| Texas Instruments Incorporated
| 1.6-GSPS, 12-bit, Analog-to-Digital Converter
| Marketing part#   ADC12QJ1600AAVQ1
| Voltage Range   1.05V - 1.15V & 1.8V - 2.0V
| Package-type   BGA
| #pins/pkg drawing   144-pin AAV
[IBIS Ver]   4.1
[File name]   adc12qj1600aav.ibs
[File Rev]   1.0
[Date]   12/15/2021
[Source]   Model built from spectre simulations at:
   Texas Instruments Incorporated.
   12500 TI Blvd
   Dallas, TX -75243
   Support: https://e2e.ti.com/support/data-converters/f/data-converters-forum
[Notes]   Rev 1.0: 12/15/2021
[Disclaimer]  This model is designed as an aid for customers of Texas Instruments
 TI and its licensors and suppliers make no warranties, either expressed
 or implied, with respect to this  model, including the warranties of
 merchantability or fitness for a particular purpose.
 The model is provided solely on an "as is" basis. The entire risk as to
 its quality and performance is with the customer.
[Copyright] (C)Copyright 2021 Texas Instruments Incorporated.
   All rights reserved.
[Component]   ADC12QJ1600AAVQ1_PECL   | PECL input on SYNCB, DEVCLK, SYSREF
[Manufacturer]  Texas Instruments Incorporated
[Package]   |144-pin BGA AAV package
|   typ   min   max
R_pkg   0.160   0.009   0.397
L_pkg   1.73E-09   4.81E-10   3.76E-09
C_pkg   7.00E-13   1.77E-13   1.64E-12
[Pin]   signal_name  model_name   R_pin   L_pin   C_pin
A1   AGND   GND
A2   INA+   NC   0.29421   2.39E-09   8.75E-13
A3   INA-   NC   0.29421   2.37E-09   8.77E-13
A4   AGND   GND
A5   AGND   GND
A6   INB+   NC   0.29156   2.27E-09   8.69E-13
A7   INB-   NC   0.29004   2.23E-09   8.66E-13
A8   AGND   GND
A9   CALTRIG   INPUT   0.17604   1.67E-09   5.27E-13
A10   VD11   POWER
A11   DGND   GND
A12   DGND   GND
B1   AGND   GND
B2   AGND   GND
B3   AGND   GND
B4   AGND   GND
B5   AGND   GND
B6   AGND   GND
B7   AGND   GND
B8   AGND   GND
B9   CALSTAT   OUTPUT   0.08157   1.80E-09   1.77E-13
B10   VD11   POWER
B11   DGND   GND
B12   DGND   GND
C1   TMSTP+   SYNCB_PECL   0.39654   3.22E-09   1.10E-12
C2   AGND   GND
C3   BG   NC   0.06662   9.15E-10   6.92E-13
C4   SYNCSE\   INPUT   0.12713   1.23E-09   8.40E-13
C5   AGND   GND
C6   AGND   GND
C7   CLKCFG0   INPUT   0.05783   8.20E-10   6.34E-13
C8   PLLREF_SE   INPUT   0.26767   3.76E-09   8.08E-13
C9   ORA   OUTPUT   0.12512   1.74E-09   4.33E-13
C10   DGND   GND
C11   D7+   NC   0.11238   1.27E-09   5.29E-13
C12   D3+   NC   0.15974   1.68E-09   6.21E-13
D1   TMSTP-   SYNCB_PECL   0.39553   3.09E-09   1.15E-12
D2   AGND   GND
D3   AGND   GND
D4   VA19   POWER
D5   VA19   POWER
D6   VA11   POWER
D7   CLKCFG1   INPUT   0.00903   4.81E-10   5.14E-13
D8   PLL_EN   INPUT   0.16984   2.55E-09   6.19E-13
D9   ORB   OUTPUT   0.05495   1.15E-09   2.51E-13
D10   VD11   POWER
D11   D7-   NC   0.11401   1.31E-09   5.25E-13
D12   D3-   NC   0.16105   1.71E-09   6.11E-13
E1   AGND   GND
E2   AGND   GND
E3   VA11   POWER
E4   AGND   GND
E5   VA11   POWER
E6   VA19   POWER
E7   AGND   GND
E8   SCS\   INPUT_PU   0.12924   1.74E-09   6.18E-13
E9   ORC   OUTPUT   0.17039   2.54E-09   4.96E-13
E10   VD11   POWER
E11   D6+   NC   0.10585   1.24E-09   5.15E-13
E12   D2+   NC   0.17042   1.72E-09   6.38E-13
F1   CLK+   DEVCLK_PECL   0.30857   2.59E-09   1.02E-12
F2   SE_CLK   INPUT   0.05749   1.43E-09   1.64E-12
F3   VA11   POWER
F4   AGND   GND
F5   VA11   POWER
F6   VA19   POWER
F7   AGND   GND
F8   SCLK   INPUT   0.06994   1.23E-09   5.56E-13
F9   ORD   OUTPUT   0.10254   1.74E-09   4.79E-13
F10   DGND   GND
F11   D6-   NC   0.10617   1.32E-09   5.12E-13
F12   D2-   NC   0.17077   1.77E-09   6.34E-13
G1   CLK-   DEVCLK_PECL   0.30912   2.61E-09   1.00E-12
G2   SE_GND   GND   0.05431   1.31E-09   1.58E-12
G3   VA11   POWER
G4   AGND   GND
G5   VA11   POWER
G6   VA19   POWER
G7   AGND   GND
G8   SDI   INPUT   0.04691   9.40E-10   6.68E-13
G9   SDO   OUTPUT   0.1   1.53E-09   5.24E-13
G10   DGND   GND
G11   D5+   NC   0.09799   1.20E-09   4.90E-13
G12   D1+   NC   0.16586   1.74E-09   6.24E-13
H1   AGND   GND
H2   AGND   GND
H3   VA11   POWER
H4   AGND   GND
H5   VA11   POWER
H6   VA19   POWER
H7   AGND   GND
H8   VD11   POWER
H9   VD11   POWER
H10   VD11   POWER
H11   D5-   NC   0.10149   1.24E-09   4.91E-13
H12   D1-   NC   0.16843   1.81E-09   6.24E-13
J1   SYSREF+   SYSREF_PECL   0.29068   2.61E-09   9.76E-13
J2   AGND   GND
J3   PGND   GND
J4   VPLL19   POWER
J5   VPLL19   POWER
J6   VA11   POWER
J7   PLLREFO+   LVDSP_MODE_0_V1P8   0.00902   4.91E-10   4.99E-13
J8   VTRIG   POWER
J9   TRIGOUT+   LVDSP   0.06885   9.55E-10   6.39E-13
J10   VD11   POWER
J11   D4+   NC   0.12851   1.35E-09   5.52E-13
J12   D0+   NC   0.17935   1.78E-09   6.56E-13
K1   SYSREF-   SYSREF_PECL   0.28925   2.55E-09   9.73E-13
K2   AGND   GND
K3   TDIODE+   NC   0.05067   1.14E-09   8.01E-13
K4   TDIODE-   NC   0.04958   1.12E-09   7.88E-13
K5   PGND   GND
K6   VREFO   POWER
K7   PLLREFO-   LVDSN_MODE_0_V1P8   0.00927   5.06E-10   5.46E-13
K8   VTRIG   POWER
K9   TRIGOUT-   LVDSN   0.07317   1.04E-09   6.64E-13
K10   DGND   GND
K11   D4-   NC   0.133   1.46E-09   5.57E-13
K12   D0-   NC   0.18263   1.86E-09   6.52E-13
L1   AGND   GND
L2   AGND   GND
L3   AGND   GND
L4   AGND   GND
L5   AGND   GND
L6   AGND   GND
L7   AGND   GND
L8   AGND   GND
L9   DGND   GND
L10   VD11   POWER
L11   DGND   GND
L12   DGND   GND
M1   AGND   GND
M2   IND+   NC   0.29422   2.39E-09   8.76E-13
M3   IND-   NC   0.29417   2.37E-09   8.75E-13
M4   AGND   GND
M5   AGND   GND
M6   INC+   NC   0.29159   2.49E-09   8.64E-13
M7   INC-   NC   0.29018   2.45E-09   8.64E-13
M8   AGND   GND
M9   PD   INPUT   0.15035   1.56E-09   4.67E-13
M10   VD11   POWER
M11   DGND   GND
M12   DGND   GND
[Diff pin]  inv_pin  vdiff  tdelay_typ  tdelay_min  tdelay_max
A2   A3   0.0   0.0s   0.0s   0.0s   | INA
A6   A7   0.0   0.0s   0.0s   0.0s   | INB
M2   M3   0.0   0.0s   0.0s   0.0s   | IND
M6   M7   0.0   0.0s   0.0s   0.0s   | INC
C1   D1   0.0   0.0s   0.0s   0.0s   | TMSTP
F1   G1   0.0   0.0s   0.0s   0.0s   | CLK
J1   K1   0.0   0.0s   0.0s   0.0s   | SYSREF
J7   K7   0.0   0.0s   0.0s   0.0s   | PLLREFO, LVDS output
J9   K9   0.0   0.0s   0.0s   0.0s   | TRIGOUT, LVDS output
J12   K12   0.0   0.0s   0.0s   0.0s   | D0 output
G12   H12   0.0   0.0s   0.0s   0.0s   | D1 output
E12   F12   0.0   0.0s   0.0s   0.0s   | D2 output
C12   D12   0.0   0.0s   0.0s   0.0s   | D3 output
J11   K11   0.0   0.0s   0.0s   0.0s   | D4 output
G11   H11   0.0   0.0s   0.0s   0.0s   | D5 output
E11   F11   0.0   0.0s   0.0s   0.0s   | D6 output
C11   D11   0.0   0.0s   0.0s   0.0s   | D7 output
[Component]   ADC12QJ1600AAVQ1_LVDS   | 100 Ohm termination on SYNCB, DEVCLK, SYSREF
[Manufacturer]  Texas Instruments Incorporated
[Package]   |144-pin BGA AAV package
|   typ   min   max
R_pkg   0.160   0.009   0.397
L_pkg   1.73E-09   4.81E-10   3.76E-09
C_pkg   7.00E-13   1.77E-13   1.64E-12
[Pin]   signal_name  model_name   R_pin   L_pin   C_pin
A1   AGND   GND
A2   INA+   NC   0.29421   2.39E-09   8.75E-13
A3   INA-   NC   0.29421   2.37E-09   8.77E-13
A4   AGND   GND
A5   AGND   GND
A6   INB+   NC   0.29156   2.27E-09   8.69E-13
A7   INB-   NC   0.29004   2.23E-09   8.66E-13
A8   AGND   GND
A9   CALTRIG   INPUT   0.17604   1.67E-09   5.27E-13
A10   VD11   POWER
A11   DGND   GND
A12   DGND   GND
B1   AGND   GND
B2   AGND   GND
B3   AGND   GND
B4   AGND   GND
B5   AGND   GND
B6   AGND   GND
B7   AGND   GND
B8   AGND   GND
B9   CALSTAT   OUTPUT   0.08157   1.80E-09   1.77E-13
B10   VD11   POWER
B11   DGND   GND
B12   DGND   GND
C1   TMSTP+   SYNCB_LVDS   0.39654   3.22E-09   1.10E-12
C2   AGND   GND
C3   BG   NC   0.06662   9.15E-10   6.92E-13
C4   SYNCSE\   INPUT   0.12713   1.23E-09   8.40E-13
C5   AGND   GND
C6   AGND   GND
C7   CLKCFG0   INPUT   0.05783   8.20E-10   6.34E-13
C8   PLLREF_SE   INPUT   0.26767   3.76E-09   8.08E-13
C9   ORA   OUTPUT   0.12512   1.74E-09   4.33E-13
C10   DGND   GND
C11   D7+   NC   0.11238   1.27E-09   5.29E-13
C12   D3+   NC   0.15974   1.68E-09   6.21E-13
D1   TMSTP-   SYNCB_LVDS   0.39553   3.09E-09   1.15E-12
D2   AGND   GND
D3   AGND   GND
D4   VA19   POWER
D5   VA19   POWER
D6   VA11   POWER
D7   CLKCFG1   INPUT   0.00903   4.81E-10   5.14E-13
D8   PLL_EN   INPUT   0.16984   2.55E-09   6.19E-13
D9   ORB   OUTPUT   0.05495   1.15E-09   2.51E-13
D10   VD11   POWER
D11   D7-   NC   0.11401   1.31E-09   5.25E-13
D12   D3-   NC   0.16105   1.71E-09   6.11E-13
E1   AGND   GND
E2   AGND   GND
E3   VA11   POWER
E4   AGND   GND
E5   VA11   POWER
E6   VA19   POWER
E7   AGND   GND
E8   SCS\   INPUT_PU   0.12924   1.74E-09   6.18E-13
E9   ORC   OUTPUT   0.17039   2.54E-09   4.96E-13
E10   VD11   POWER
E11   D6+   NC   0.10585   1.24E-09   5.15E-13
E12   D2+   NC   0.17042   1.72E-09   6.38E-13
F1   CLK+   DEVCLK_LVDS   0.30857   2.59E-09   1.02E-12
F2   SE_CLK   INPUT   0.05749   1.43E-09   1.64E-12
F3   VA11   POWER
F4   AGND   GND
F5   VA11   POWER
F6   VA19   POWER
F7   AGND   GND
F8   SCLK   INPUT   0.06994   1.23E-09   5.56E-13
F9   ORD   OUTPUT   0.10254   1.74E-09   4.79E-13
F10   DGND   GND
F11   D6-   NC   0.10617   1.32E-09   5.12E-13
F12   D2-   NC   0.17077   1.77E-09   6.34E-13
G1   CLK-   DEVCLK_LVDS   0.30912   2.61E-09   1.00E-12
G2   SE_GND   GND   0.05431   1.31E-09   1.58E-12
G3   VA11   POWER
G4   AGND   GND
G5   VA11   POWER
G6   VA19   POWER
G7   AGND   GND
G8   SDI   INPUT   0.04691   9.40E-10   6.68E-13
G9   SDO   OUTPUT   0.1   1.53E-09   5.24E-13
G10   DGND   GND
G11   D5+   NC   0.09799   1.20E-09   4.90E-13
G12   D1+   NC   0.16586   1.74E-09   6.24E-13
H1   AGND   GND
H2   AGND   GND
H3   VA11   POWER
H4   AGND   GND
H5   VA11   POWER
H6   VA19   POWER
H7   AGND   GND
H8   VD11   POWER
H9   VD11   POWER
H10   VD11   POWER
H11   D5-   NC   0.10149   1.24E-09   4.91E-13
H12   D1-   NC   0.16843   1.81E-09   6.24E-13
J1   SYSREF+   SYSREF_LVDS   0.29068   2.61E-09   9.76E-13
J2   AGND   GND
J3   PGND   GND
J4   VPLL19   POWER
J5   VPLL19   POWER
J6   VA11   POWER
J7   PLLREFO+   LVDSP_MODE_0_V1P8  0.00902   4.91E-10   4.99E-13
J8   VTRIG   POWER
J9   TRIGOUT+   LVDSP   0.06885   9.55E-10   6.39E-13
J10   VD11   POWER
J11   D4+   NC   0.12851   1.35E-09   5.52E-13
J12   D0+   NC   0.17935   1.78E-09   6.56E-13
K1   SYSREF-   SYSREF_LVDS   0.28925   2.55E-09   9.73E-13
K2   AGND   GND
K3   TDIODE+   NC   0.05067   1.14E-09   8.01E-13
K4   TDIODE-   NC   0.04958   1.12E-09   7.88E-13
K5   PGND   GND
K6   VREFO   POWER
K7   PLLREFO-   LVDSN_MODE_0_V1P8   0.00927   5.06E-10   5.46E-13
K8   VTRIG   POWER
K9   TRIGOUT-   LVDSN   0.07317   1.04E-09   6.64E-13
K10   DGND   GND
K11   D4-   NC   0.133   1.46E-09   5.57E-13
K12   D0-   NC   0.18263   1.86E-09   6.52E-13
L1   AGND   GND
L2   AGND   GND
L3   AGND   GND
L4   AGND   GND
L5   AGND   GND
L6   AGND   GND
L7   AGND   GND
L8   AGND   GND
L9   DGND   GND
L10   VD11   POWER
L11   DGND   GND
L12   DGND   GND
M1   AGND   GND
M2   IND+   NC   0.29422   2.39E-09   8.76E-13
M3   IND-   NC   0.29417   2.37E-09   8.75E-13
M4   AGND   GND
M5   AGND   GND
M6   INC+   NC   0.29159   2.49E-09   8.64E-13
M7   INC-   NC   0.29018   2.45E-09   8.64E-13
M8   AGND   GND
M9   PD   INPUT   0.15035   1.56E-09   4.67E-13
M10   VD11   POWER
M11   DGND   GND
M12   DGND   GND
[Diff pin]  inv_pin  vdiff  tdelay_typ  tdelay_min  tdelay_max
A2   A3   0.0   0.0s   0.0s   0.0s   | INA
A6   A7   0.0   0.0s   0.0s   0.0s   | INB
M2   M3   0.0   0.0s   0.0s   0.0s   | IND
M6   M7   0.0   0.0s   0.0s   0.0s   | INC
C1   D1   0.0   0.0s   0.0s   0.0s   | TMSTP
F1   G1   0.0   0.0s   0.0s   0.0s   | CLK
J1   K1   0.0   0.0s   0.0s   0.0s   | SYSREF
J7   K7   0.0   0.0s   0.0s   0.0s   | PLLREFO, LVDS output
J9   K9   0.0   0.0s   0.0s   0.0s   | TRIGOUT, LVDS output
J12   K12   0.0   0.0s   0.0s   0.0s   | D0 output
G12   H12   0.0   0.0s   0.0s   0.0s   | D1 output
E12   F12   0.0   0.0s   0.0s   0.0s   | D2 output
C12   D12   0.0   0.0s   0.0s   0.0s   | D3 output
J11   K11   0.0   0.0s   0.0s   0.0s   | D4 output
G11   H11   0.0   0.0s   0.0s   0.0s   | D5 output
E11   F11   0.0   0.0s   0.0s   0.0s   | D6 output
C11   D11   0.0   0.0s   0.0s   0.0s   | D7 output
[Series Pin Mapping]   pin_2   model_name   function_table_group
C1   D1   100_Ohm   | SYNCB with 100 Ohm termination
F1   G1   100_Ohm   | DEVCLK with 100 Ohm termination
J1   K1   100_Ohm   | SYSREF with 100 Ohm termination
[Model Selector] LVDSP
LVDSP_MODE_0_V1P8   LVDS non-inverting output mode 0, buffer supply VDD1P8
LVDSP_MODE_0_V1P1   LVDS non-inverting output mode 0, buffer supply VDD1P1
[Model Selector] LVDSN
LVDSN_MODE_0_V1P8   LVDS inverting output mode 0, buffer supply VDD1P1
LVDSN_MODE_0_V1P1   LVDS inverting output mode 0, buffer supply VDD1P8
[Model] 100_Ohm
Model_type Series
Polarity Non-Inverting
Enable Active-High
|   typ   min   max
C_comp   0   0   0
[Voltage Range]   1.10V   1.05V   1.15V
[Temperature Range]  25   125   -40
[R Series]   100   80   120
| Models and submodels in the file (14): LVDSP_MODE_0_V1P8 (3-state), LVDSP_MODE_0_V1P1 (3-state), LVDSN_MODE_0_V1P8 (3-state), LVDSN_MODE_0_V1P1 (3-state), SYNCB_LVDS (Input), SYNCB_PECL (Input), DEVCLK_LVDS (Input), DEVCLK_PECL (Input), SYSREF_LVDS (Input), SYSREF_PECL (Input), INPUT (Input), INPUT_PU (Input), OUTPUT (3-state), 100_Ohm (Series)
